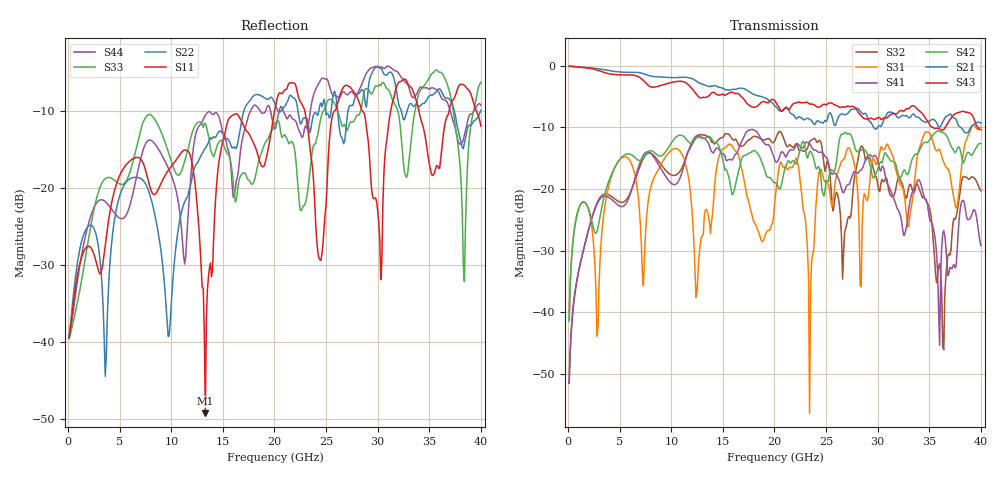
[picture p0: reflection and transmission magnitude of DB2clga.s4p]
! ADC12DJ3200QML-SP
! 196-pin ZMX package
! CLGA Ceramic Package without columns (ceramic land grid array)
! Texas Instruments 4/21/2021
! Single-ended  S-parameters
! PORT#  PORT_NAME  NET_NAME
! PORT1:  DAxN.DIEBUMP DAxN
! PORT2:  DAxN.BGA  DAxN
! PORT3:  DAxP.DIEBUMP DAxP
! PORT4:  DAxP.BGA  DAxP
! Touchstone Ver. 1.0
! Number of ports is 4
# Hz	S	MA	R	50.000000
! SCATTERING PARAMETERS  :
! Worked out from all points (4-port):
!   400 points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, 100 MHz to 40 GHz, reference 50 ohm
!   strongest paths, dB at 100 MHz, 10.1 GHz, 20.1 GHz, 30.1 GHz, 40 GHz:
!     S43: -0.1, -2.7, -5.9, -8.4, -10.4
!     S21: -0.1, -2.0, -6.6, -9.8, -9.3
!     S42: -41.4, -12.3, -19.0, -16.3, -12.7
!     S41: -51.5, -19.2, -15.6, -16.0, -29.2
!     S31: -41.4, -13.6, -20.9, -14.9, -10.0
!     S32: -51.5, -17.8, -11.9, -20.2, -20.3
!   lowest |S11| = -49.3 dB at 13.3 GHz (marker M1), VSWR 1.01, Z = 49.8 - j0.252 ohm
!   |S11| at or under -10 dB: start of sweep to 20 GHz; 22.93 GHz to 25.84 GHz (2.908 GHz wide, 11.9 % of centre); 33.99 GHz to 36.92 GHz (2.928 GHz wide, 8.26 % of centre)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
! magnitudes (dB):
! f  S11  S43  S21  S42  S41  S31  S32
! 100 MHz  -39.5  -0.1  -0.1  -41.4  -51.5  -41.4  -51.5
! 11.5 GHz  -15.1  -2.9  -1.9  -12.0  -14.6  -16.8  -14.5
! 13.3 GHz  -49.3  -5.2  -3.2  -11.7  -11.9  -23.4  -11.3
! 22.2 GHz  -7.5  -6.0  -8.6  -15.6  -12.6  -15.3  -12.9
! 23.4 GHz  -14.4  -6.2  -8.7  -13.9  -12.6  -56.4  -12.3
! 24.4 GHz  -29.4  -6.7  -9.2  -16.9  -14.0  -16.9  -12.1
! 40 GHz  -12.0  -10.4  -9.3  -12.7  -29.2  -10.0  -20.3
